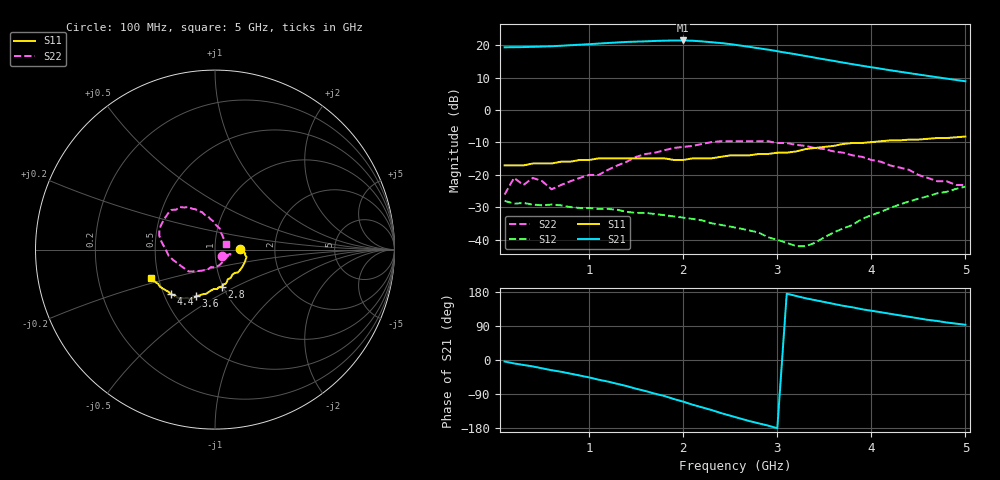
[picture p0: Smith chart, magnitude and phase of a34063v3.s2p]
!  INA-34063  S PARAMETERS
!  Vd = 3 V  LAST UPDATED 04-16-98
# ghz s ma r 50
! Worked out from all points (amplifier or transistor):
!   50 points, 100 MHz to 5 GHz, reference 50 ohm
!   highest |S21| = 21.4 dB at 2 GHz (marker M1)
!   |S21| within 3 dB of that: start of sweep to 2.936 GHz
!   unconditionally stable (mu >= 1): start of sweep to end of sweep
!   at 900 MHz: K = 1.68, MAG = 20.3 dB, |S12| = -30.2 dB
!   at 2.6 GHz: K = 2.95, MAG = 20.6 dB, |S12| = -36.5 dB
!   at 5 GHz: K = 2.37, MAG = 9.7 dB, |S12| = -23.6 dB
!   S11 on the Smith chart (normalised r, x): 100 MHz: 1.33, +0.01; 2.8 GHz: 0.99, -0.43; 3.6 GHz: 0.72, -0.40; 4.4 GHz: 0.54, -0.31; 5 GHz: 0.45, -0.17
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0.1  0.14 2.0  9.23 -4.0  0.04 1.6  0.05 -42.0
0.2  0.14 3.0  9.26 -9.0  0.036 -1.0  0.09 -24.0
0.7  0.16 -3.0  9.75 -31.0  0.034 -14.0  0.07 -44.0
1  0.17 -10.0  10.31 -46.0  0.031 -15.0  0.1 -90.0
1.2  0.18 -16.0  10.75 -57.0  0.03 -19.0  0.12 -111.0
1.4  0.18 -23.0  11.16 -69.0  0.027 -20.0  0.16 -131.0
1.6  0.18 -32.0  11.39 -82.0  0.026 -22.0  0.21 -154.0
1.8  0.18 -45.0  11.68 -95.0  0.024 -27.0  0.24 -166.0
2  0.17 -55.0  11.76 -110.0  0.022 -30.0  0.27 -178.0
2.1  0.18 -61.0  11.65 -118.0  0.021 -34.0  0.28 178.0
2.2  0.18 -64.0  11.37 -125.0  0.02 -36.0  0.3 172.0
2.4  0.19 -69.0  10.73 -140.0  0.017 -43.0  0.33 160.0
2.6  0.2 -74.0  9.85 -154.0  0.015 -54.0  0.33 152.0
2.8  0.21 -79.0  8.92 -167.0  0.013 -73.0  0.33 142.0
3  0.22 -87.0  8.03 -180.0  0.01 -96.0  0.31 134.0
3.3  0.25 -101.0  6.78 163.0  0.008 -143.0  0.28 122.0
3.4  0.26 -106.0  6.39 158.0  0.009 -153.0  0.26 119.0
3.6  0.28 -112.0  5.69 148.0  0.013 -172.0  0.23 112.0
3.9  0.31 -120.0  4.8 134.0  0.021 174.0  0.19 102.0
4.2  0.34 -128.0  4.09 122.0  0.031 163.0  0.14 89.0
4.4  0.35 -135.0  3.7 114.0  0.039 156.0  0.12 77.0
5  0.39 -156.0  2.77 93.0  0.066 141.0  0.07 24.0
